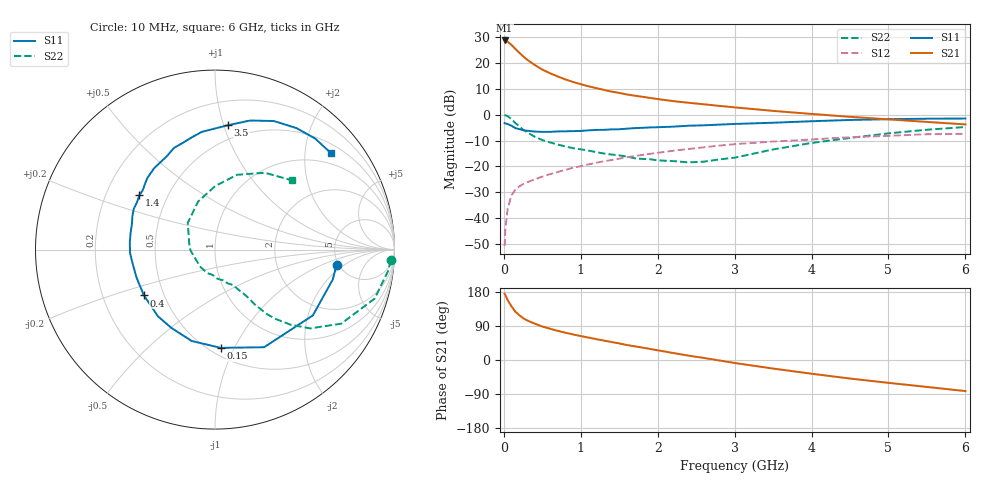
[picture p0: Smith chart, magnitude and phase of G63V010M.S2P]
! SIEMENS Small Signal Semiconductors
! BFG193
! Si NPN RF Bipolar Junction Transistor in SOT223
! VCE = 3 V  IC = 10 mA
! Common Emitter S-Parameters:  August  1996
# GHz  S  MA  R  50
!  f  S11  S21  S12  S22
! GHz  MAG  ANG  MAG  ANG  MAG  ANG  MAG  ANG
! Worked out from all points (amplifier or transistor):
!   36 points, 10 MHz to 6 GHz, reference 50 ohm
!   highest |S21| = 28.6 dB at 10 MHz (marker M1)
!   |S21| within 3 dB of that: start of sweep to 140.8 MHz
!   unconditionally stable (mu >= 1): 886.8 MHz to 2.565 GHz
!   at 250 MHz: K = 0.54, MSG = 24.7 dB, |S12| = -26.8 dB
!   at 1.4 GHz: K = 1.07, MAG = 11.6 dB, |S12| = -17.5 dB
!   at 6 GHz: K = 0.88, MSG = 1.8 dB, |S12| = -7.4 dB
!   S11 on the Smith chart (normalised r, x): 10 MHz: 4.81, -1.52; 150 MHz: 0.57, -0.88; 400 MHz: 0.39, -0.25; 1.4 GHz: 0.35, +0.29; 3.5 GHz: 0.38, +1.03; 6 GHz: 0.71, +2.61
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0.01  0.6829 -7.1  26.92 175.1  0.0029 87.6  0.9817 -3.5
0.02  0.6768 -14.3  26.85 171.5  0.0063 85.7  0.9716 -7.1
0.05  0.6571 -33.9  25.47 157.8  0.0154 74.2  0.9301 -17.1
0.1  0.6088 -63.3  22.06 141.5  0.0279 64.8  0.8154 -30.4
0.15  0.5484 -86.7  18.44 127.4  0.0357 56.2  0.6888 -39.6
0.2  0.5254 -104.3  15.66 118.3  0.0411 53.4  0.5941 -44.8
0.25  0.4996 -119.0  13.34 110.6  0.0457 50.6  0.5137 -48.8
0.3  0.4892 -130.5  11.57 104.7  0.0494 50.0  0.459 -51.3
0.4  0.4711 -147.2  9.083 96.0  0.0563 49.5  0.3748 -54.1
0.5  0.4642 -160.2  7.389 88.3  0.0635 49.6  0.3234 -55.5
0.6  0.4652 -169.8  6.273 82.5  0.071 50.1  0.2908 -57.1
0.7  0.4738 -177.8  5.438 76.9  0.0782 50.5  0.2648 -59.2
0.9  0.4796 168.7  4.263 67.5  0.0944 49.9  0.2256 -62.3
1.1  0.4967 157.9  3.517 59.2  0.1094 49.0  0.2023 -69.0
1.4  0.5186 144.3  2.777 47.4  0.1329 45.6  0.1698 -79.7
1.7  0.5485 133.5  2.317 36.1  0.1586 41.8  0.1439 -93.7
2.2  0.5853 117.3  1.821 18.6  0.2007 32.8  0.1268 -128.3
2.8  0.6411 101.0  1.473 -1.2  0.2522 20.9  0.1366 -178.4
3.5  0.697 84.0  1.179 -22.6  0.3021 4.8  0.2129 135.4
4.5  0.7879 65.4  0.906 -48.9  0.3663 -15.0  0.3547 89.7
5.5  0.833 48.0  0.723 -71.1  0.4183 -39.1  0.5105 57.0
6  0.8409 39.6  0.647 -82.0  0.4247 -53.0  0.5767 42.0
